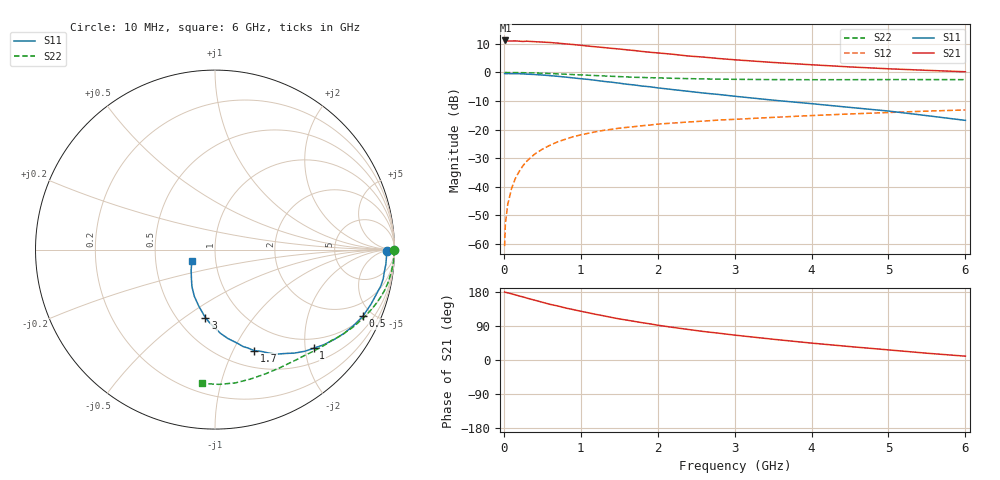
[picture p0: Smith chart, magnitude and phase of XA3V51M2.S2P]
! SIEMENS Discrete & RF Semiconductors
! BFY180
! Si NPN RF Bipolar Junction Transistor in MICRO-X
! VCE = 3.5 V  IC = 1.2 mA
! Common Emitter S-Parameters:  May  1997
# GHz  S  MA  R  50
!  f  S11  S21  S12  S22
! GHz  MAG  ANG  MAG  ANG  MAG  ANG  MAG  ANG
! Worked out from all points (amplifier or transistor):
!   36 points, 10 MHz to 6 GHz, reference 50 ohm
!   highest |S21| = 11.2 dB at 20 MHz (marker M1)
!   |S21| within 3 dB of that: start of sweep to 1.499 GHz
!   unconditionally stable (mu >= 1): 3.575 GHz to end of sweep
!   at 250 MHz: K = 0.09, MSG = 21.8 dB, |S12| = -32.7 dB
!   at 1.4 GHz: K = 0.54, MSG = 14.2 dB, |S12| = -19.9 dB
!   at 6 GHz: K = 1.06, MAG = 5.2 dB, |S12| = -13.1 dB
!   S11 on the Smith chart (normalised r, x): 10 MHz: 44, -7; 500 MHz: 1.09, -4.39; 1 GHz: 0.78, -2.18; 1.7 GHz: 0.68, -1.21; 3 GHz: 0.68, -0.61; 6 GHz: 0.77, -0.10
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0.01  0.9569 -0.4  3.552 179.4  0.0009 84.2  0.9969 -0.2
0.02  0.954 -0.9  3.645 178.6  0.0022 87.5  0.9999 -0.6
0.05  0.9562 -2.4  3.57 177.3  0.0048 86.6  0.9974 -1.4
0.1  0.9553 -4.9  3.569 174.7  0.0092 86.7  0.9964 -2.8
0.15  0.9515 -7.6  3.585 171.9  0.0139 84.3  0.9962 -4.2
0.25  0.9457 -12.4  3.505 166.5  0.0233 81.5  0.9916 -7.1
0.3  0.9357 -14.7  3.538 163.3  0.028 79.8  0.9871 -8.4
0.5  0.9033 -24.3  3.413 152.4  0.0451 73.2  0.971 -13.7
0.6  0.8802 -28.8  3.358 146.9  0.053 70.7  0.9589 -16.2
0.8  0.8307 -37.2  3.174 137.4  0.0675 64.6  0.9332 -20.9
1  0.7774 -45.0  2.998 128.7  0.0805 59.6  0.9072 -25.3
1.1  0.7554 -48.6  2.899 124.5  0.086 57.3  0.8943 -27.2
1.4  0.6755 -59.6  2.652 112.3  0.1009 51.4  0.8581 -32.9
1.7  0.6039 -68.8  2.424 101.8  0.1126 46.7  0.8241 -37.8
2  0.5376 -76.4  2.204 91.8  0.1245 42.8  0.8045 -42.3
2.2  0.5009 -81.7  2.085 86.0  0.1297 40.4  0.791 -45.2
2.6  0.4355 -90.2  1.86 75.1  0.1406 36.6  0.7707 -50.4
3  0.3833 -98.0  1.671 65.7  0.1508 33.1  0.7585 -55.5
3.5  0.3271 -106.1  1.499 54.8  0.1633 29.4  0.7506 -61.7
4.5  0.2441 -121.7  1.252 35.4  0.1874 21.9  0.7477 -74.6
5.5  0.175 -139.4  1.091 17.9  0.2102 14.3  0.7511 -88.4
6  0.1447 -152.9  1.03 10.1  0.2204 10.0  0.7491 -95.4
